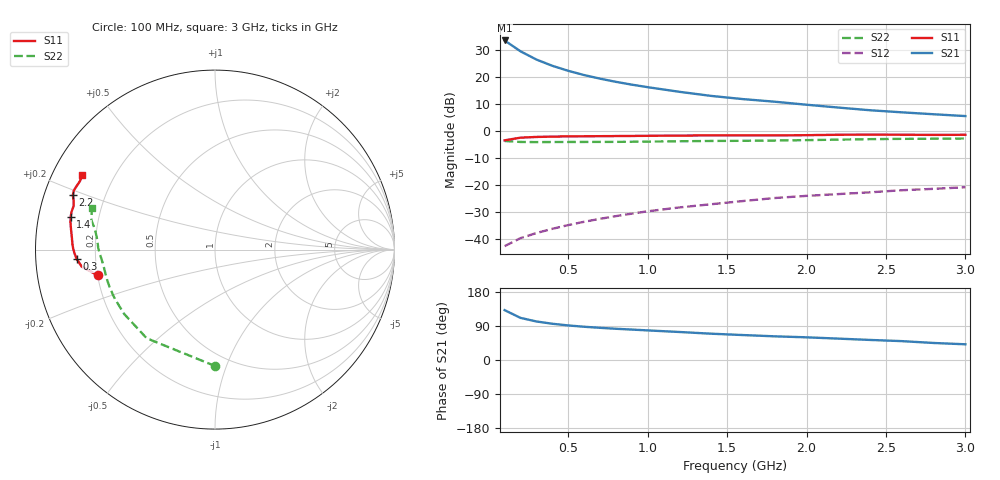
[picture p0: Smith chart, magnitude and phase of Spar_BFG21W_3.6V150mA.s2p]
! Filename: 3_6150bfg21.001
! Title: BFG21W
! Bias: Vce=3.6V; Ic=150mA
! Company: NXP Semiconductors NL
! User: Quality&Reliability T&D
! Measure time: 10 Nov 1999 / 11:44:50
#  MHz  S  MA  R 50
! Freq  S11  S21  S12  S22  :
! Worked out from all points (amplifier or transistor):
!   20 points, 100 MHz to 3 GHz, reference 50 ohm
!   highest |S21| = 33.5 dB at 100 MHz (marker M1)
!   |S21| within 3 dB of that: start of sweep to 174.6 MHz
!   unconditionally stable (mu >= 1): 591.4 MHz to end of sweep
!   at 400 MHz: K = 0.92, MSG = 30.2 dB, |S12| = -36.3 dB
!   at 1.2 GHz: K = 1.06, MAG = 19.9 dB, |S12| = -28.4 dB
!   at 3 GHz: K = 1.05, MAG = 11.8 dB, |S12| = -20.9 dB
!   S11 on the Smith chart (normalised r, x): 100 MHz: 0.20, -0.10; 300 MHz: 0.13, -0.03; 1.4 GHz: 0.10, +0.11; 2.2 GHz: 0.08, +0.18; 3 GHz: 0.09, +0.26
100  0.6682 -167.6  47.39 131.6  0.00731 57.9  0.6494 -89.8
200  0.7485 -172.7  29.83 111.1  0.0103 55.6  0.6236 -127.6
300  0.7723 -176.1  21 101.7  0.01279 59.5  0.6201 -144.5
400  0.7835 -178.6  16.08 95.7  0.01533 63.0  0.6219 -153.8
500  0.7907 179.5  12.99 91.2  0.01796 65.5  0.6233 -159.8
600  0.795 177.8  10.83 87.8  0.02068 67.7  0.6241 -164.0
700  0.7981 176.2  9.298 84.9  0.02347 69.3  0.6245 -167.2
800  0.8018 174.6  8.114 82.4  0.02632 70.7  0.6259 -170.0
900  0.8059 173.2  7.196 80.3  0.02928 72.0  0.629 -172.4
1000  0.8105 171.9  6.459 78.1  0.03236 72.5  0.6329 -174.5
1200  0.8192 169.4  5.299 73.9  0.03816 73.2  0.6424 -178.0
1400  0.8245 167.4  4.448 69.4  0.04374 73.3  0.6508 179.2
1600  0.8265 165.2  3.882 65.8  0.05015 73.4  0.655 176.7
1800  0.8244 162.8  3.473 62.5  0.05703 73.2  0.6627 174.0
2000  0.8329 161.0  3.054 59.8  0.06252 73.5  0.6743 171.2
2200  0.8481 159.1  2.706 56.4  0.06746 73.2  0.6885 169.0
2400  0.8525 157.3  2.413 52.9  0.07271 72.2  0.7026 167.3
2600  0.8487 155.5  2.207 49.8  0.07953 71.1  0.7119 165.8
2800  0.8435 153.2  2.034 44.9  0.08438 69.3  0.7159 163.8
3000  0.8471 150.7  1.881 41.4  0.09033 68.3  0.7227 161.3
